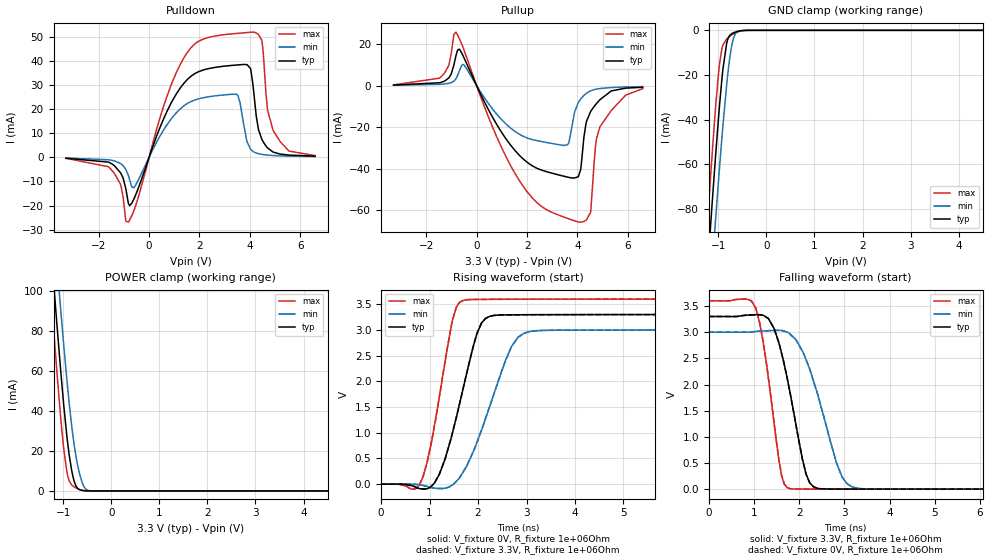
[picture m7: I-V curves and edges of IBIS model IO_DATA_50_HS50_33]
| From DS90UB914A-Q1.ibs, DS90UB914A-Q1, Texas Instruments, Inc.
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|   Model IO_DATA_50_HS50_33
[Model]  IO_DATA_50_HS50_33
Model_type   I/O
Polarity   Non-Inverting
Enable   Active-Low
Vinl =   0.8
Vinh =   2.0
Vmeas = 1.5000V
|   typ   min   max
|   (nom)   (fast)   (slow)
C_comp   0.7658pF   0.7658pF   1.107pF|
[Temperature Range]   25.0000   105.000   -40.0000
[Voltage Range]   3.3000V   3.0000V   3.6000V
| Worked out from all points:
|   slope of the pulldown table from 0 to 0.495 V, typ, clamps not added: 35.6 ohm
|   slope of the pullup table from 0 to 0.495 V, typ, clamps not added: 40.7 ohm
|   GND clamp passes 1 mA (typ) near -0.67 V on its own axis
|   POWER clamp passes 1 mA (typ) near -0.68 V on its own axis
|   falling waveform, V_fixture 3.3V, R_fixture 1e+06Ohm: 20-80 % time 454ps typ, 607ps min, 337ps max; typ from 3.3 V to 0 V
|   rising waveform, V_fixture 0V, R_fixture 1e+06Ohm: 20-80 % time 518ps typ, 680ps min, 393ps max; typ from 0 V to 3.3 V
|   rising waveform, V_fixture 3.3V, R_fixture 1e+06Ohm: 20-80 % time 518ps typ, 680ps min, 393ps max; typ from 0 V to 3.3 V
|   falling waveform, V_fixture 0V, R_fixture 1e+06Ohm: 20-80 % time 454ps typ, 607ps min, 337ps max; typ from 3.3 V to 0 V
[Pulldown]
|   Voltage   I(typ)   I(min)   I(max)
-3.3V     -398.6uA   -308.4uA   -441.5uA
-1.607V   -2.008mA   -1.038mA   -3.915mA
-1.142V   -6.34mA    -2.537mA   -11.03mA
-825mV    -19.01mA   -7.459mA   -26.88mA
-597.3mV  -17.1mA    -12.5mA    -21.91mA
1.472V    31.7mA     21.95mA    42.69mA
3.472V    38.2mA     26.05mA    51.26mA
4.125V    29.83mA    2.412mA    51.83mA
4.471V    7.548mA    1.199mA    48.51mA
4.699V    3.892mA    904.3uA    19.71mA
4.917V    2.181mA    733.2uA    11.27mA
6.59V     463.1uA    300.8uA    707.4uA
[GND Clamp]
|   Voltage   I(typ)   I(min)   I(max)
-3.3V     -797.8mA   -802.3mA   -798.9mA
-1.231V   -109.3mA   -136.9mA   -87.72mA
-1.201V   -99.97mA   -127.8mA   -78.2mA
-1.122V   -75.61mA   -104mA     -53.52mA
-1.073V   -60.86mA   -89.38mA   -38.97mA
-983.4mV  -35.94mA   -63.89mA   -16.79mA
-904.2mV  -17.38mA   -42.71mA   -6.495mA
-815.1mV  -4.825mA   -22.04mA   -3.687mA
-735.9mV  -1.733mA   -8.725mA   -2.326mA
-676.5mV  -1.028mA   -3.116mA   -1.513mA
-409.2mV  -15.42uA   -13.48uA   -30.67uA
6.59V     0A         0A         0A
[Pullup]
|   Voltage   I(typ)   I(min)   I(max)
-3.3V     325uA      225.8uA    411.8uA
-1.468V   1.438mA    671.4uA    3.669mA
-825mV    14.44mA    3.308mA    25.83mA
-508.2mV  13.57mA    10.06mA    17.31mA
1.739V    -34mA      -23.65mA   -46.49mA
3.61V     -43.98mA   -28.38mA   -63.84mA
4.125V    -40.43mA   -6.45mA    -65.66mA
4.333V    -18.57mA   -3.808mA   -64.75mA
4.521V    -12.43mA   -2.449mA   -60.87mA
4.709V    -9.237mA   -1.735mA   -29.82mA
4.897V    -6.664mA   -1.33mA    -19.66mA
6.59V     -713.8uA   -421.6uA   -1.399mA
[POWER Clamp]
|   Voltage   I(typ)   I(min)   I(max)
-3.3V     802.5mA    808.9mA    802mA
-1.31V    139.8mA    168.7mA    117.3mA
-1.231V   114.8mA    144.4mA    91.52mA
-1.211V   108.6mA    138.4mA    85.16mA
-1.132V   84.2mA     114.6mA    60.34mA
-1.082V   69.45mA    100mA      45.61mA
-924mV    27.79mA    56.17mA    9.883mA
-795.3mV  7.174mA    27.45mA    2.45mA
-656.7mV  613.2uA    8.486mA    694.4uA
-547.8mV  99.32uA    1.452mA    115.9uA
-409.2mV  3.688uA    30.95uA    3.022uA
6.59V     0A         0A         0A
[Ramp]
R_load = 1e+06
|   typ   min   max
dV/dt_r   1.97978/5.1816e-10   1.79965/6.79662e-10   2.15988/3.93384e-10
dV/dt_f   1.97979/4.53788e-10   1.79966/6.07164e-10   2.15989/3.36704e-10
[Falling Waveform]
V_fixture = 3.3V
V_fixture_min = 3V
V_fixture_max = 3.6V
R_fixture = 1e+06Ohm
C_fixture = 0F
|   Time   V(typ)   V(min)   V(max)
0s        3.3V       3V         3.6V
1.041ns   3.334V     3.014V     3.461V
1.208ns   3.321V     3.024V     2.799V
1.447ns   3.071V     3.034V     1.262V
1.611ns   2.602V     3.033V     265.3mV
1.731ns   2.145V     3.002V     33.39mV
2.235ns   121.1mV    2.294V     1.926mV
2.827ns   2.286mV    503.7mV    1.157mV
3.176ns   1.668mV    41.87mV    915uV
10.05ns   193.1uV    272.6uV    94.54uV
[Rising Waveform]
V_fixture = 0V
V_fixture_min = 0V
V_fixture_max = 0V
R_fixture = 1e+06Ohm
C_fixture = 0F
|   Time   V(typ)   V(min)   V(max)
0s        85.23uV    137.2uV    15.28uV
801.3ps   -86.42mV   -13.68mV   6.187mV
949ps     -86.52mV   -44.02mV   422.8mV
1.203ns   195.9mV    -84.71mV   1.704V
1.471ns   993.1mV    -15.88mV   3.183V
1.671ns   1.772V     202.9mV    3.566V
2.073ns   3.137V     1.054V     3.594V
2.691ns   3.293V     2.679V     3.596V
2.948ns   3.295V     2.935V     3.597V
10.05ns   3.3V       3V         3.6V
[Rising Waveform]
V_fixture = 3.3V
V_fixture_min = 3V
V_fixture_max = 3.6V
R_fixture = 1e+06Ohm
C_fixture = 0F
|   Time   V(typ)   V(min)   V(max)
0s        192.6uV    277.5uV    102.7uV
801.3ps   -85.91mV   -13.52mV   7.155mV
949ps     -85.56mV   -43.75mV   424mV
1.203ns   197.3mV    -83.83mV   1.705V
1.471ns   994.8mV    -14.38mV   3.184V
1.671ns   1.774V     204.8mV    3.566V
2.073ns   3.137V     1.056V     3.594V
2.691ns   3.293V     2.68V      3.597V
2.948ns   3.295V     2.936V     3.597V
10.05ns   3.3V       3V         3.6V
[Falling Waveform]
|Gnd
V_fixture = 0V
V_fixture_min = 0V
V_fixture_max = 0V
R_fixture = 1e+06Ohm
C_fixture = 0F
|   Time   V(typ)   V(min)   V(max)
0s        3.3V       3V         3.6V
1.041ns   3.334V     3.014V     3.46V
1.208ns   3.321V     3.024V     2.798V
1.447ns   3.07V      3.033V     1.261V
1.611ns   2.601V     3.033V     264.4mV
1.731ns   2.143V     3.002V     33.08mV
2.235ns   120.5mV    2.293V     1.791mV
2.827ns   2.096mV    502mV      1.045mV
3.176ns   1.536mV    41.36mV    810.4uV
10.05ns   85.76uV    132.5uV    7.134uV
